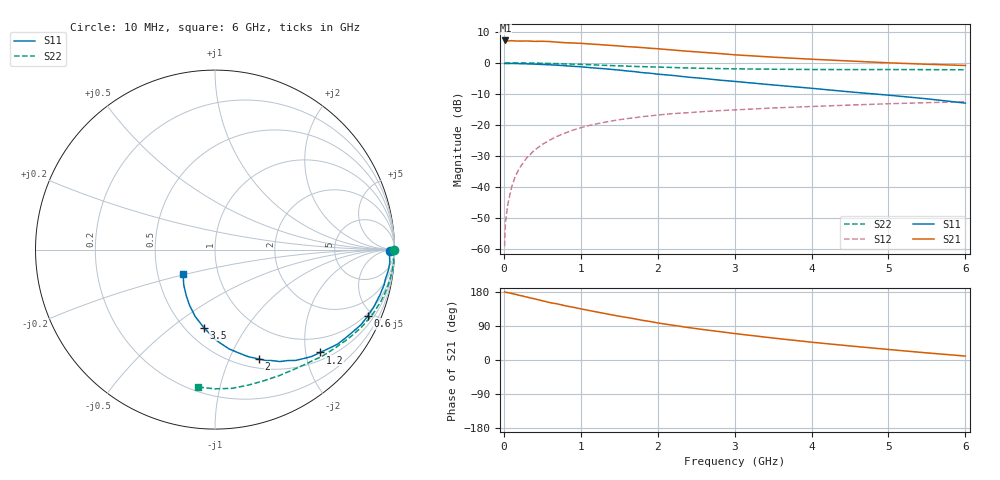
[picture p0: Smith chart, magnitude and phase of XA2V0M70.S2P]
! SIEMENS Discrete & RF Semiconductors
! BFY180
! Si NPN RF Bipolar Junction Transistor in MICRO-X
! VCE = 2 V  IC = 0.7 mA
! Common Emitter S-Parameters:  May  1997
# GHz  S  MA  R  50
!  f  S11  S21  S12  S22
! GHz  MAG  ANG  MAG  ANG  MAG  ANG  MAG  ANG
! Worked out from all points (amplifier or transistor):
!   36 points, 10 MHz to 6 GHz, reference 50 ohm
!   highest |S21| = 7.2 dB at 20 MHz (marker M1)
!   |S21| within 3 dB of that: start of sweep to 2.157 GHz
!   unconditionally stable (mu >= 1): 4.282 GHz to end of sweep
!   at 250 MHz: K = 0.06, MSG = 19.7 dB, |S12| = -32.3 dB
!   at 1.4 GHz: K = 0.46, MSG = 12.2 dB, |S12| = -18.8 dB
!   at 6 GHz: K = 1.05, MAG = 4.4 dB, |S12| = -12.5 dB
!   S11 on the Smith chart (normalised r, x): 10 MHz: 68, -17; 600 MHz: 0.87, -4.65; 1.2 GHz: 0.66, -2.30; 2 GHz: 0.60, -1.29; 3.5 GHz: 0.61, -0.66; 6 GHz: 0.68, -0.19
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0.01  0.9727 -0.4  2.266 179.7  0.0011 79.7  0.9992 -0.2
0.02  0.9727 -0.7  2.295 178.9  0.0026 86.6  0.9997 -0.5
0.05  0.9722 -1.8  2.249 177.9  0.0051 87.8  0.998 -1.3
0.1  0.9766 -3.9  2.28 175.6  0.0098 86.7  0.9948 -2.5
0.15  0.9746 -6.0  2.251 173.3  0.0148 86.5  0.9992 -3.8
0.2  0.9695 -7.9  2.246 170.7  0.0197 84.8  0.9958 -4.9
0.3  0.9626 -11.7  2.251 166.0  0.0295 81.5  0.9924 -7.4
0.4  0.9531 -15.4  2.219 161.3  0.0392 78.7  0.9892 -9.9
0.6  0.9284 -23.5  2.205 151.4  0.057 72.9  0.9761 -14.7
0.9  0.8785 -34.0  2.088 139.2  0.0821 64.7  0.9524 -21.5
1.1  0.8402 -40.9  2.021 131.0  0.0967 60.0  0.9329 -25.7
1.2  0.8203 -44.3  1.985 127.0  0.1033 57.2  0.9233 -27.9
1.5  0.7633 -54.0  1.87 115.5  0.1207 51.0  0.8936 -33.6
2  0.6568 -68.1  1.688 97.8  0.1437 42.6  0.8532 -42.0
2.2  0.6251 -72.7  1.608 91.7  0.1515 39.3  0.8407 -45.3
2.4  0.5863 -77.7  1.534 85.6  0.1569 36.7  0.8252 -48.2
2.8  0.5265 -86.1  1.412 75.0  0.1692 32.2  0.8073 -53.7
3.5  0.4395 -98.1  1.235 58.0  0.1868 25.1  0.7882 -62.9
4  0.3885 -106.5  1.143 47.0  0.1973 20.6  0.7799 -69.4
4.5  0.3394 -114.9  1.069 37.1  0.208 16.4  0.7774 -76.1
5.5  0.2625 -131.6  0.948 18.7  0.2275 8.1  0.7758 -90.0
6  0.2237 -142.6  0.906 10.4  0.2361 3.7  0.7714 -96.9
